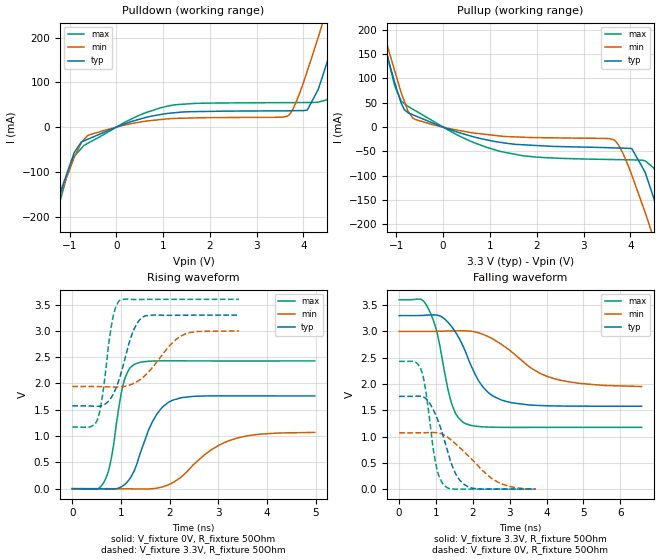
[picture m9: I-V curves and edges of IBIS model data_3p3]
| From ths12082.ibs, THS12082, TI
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|   data_3p3 Model
[Model]   data_3p3
Model_type   Output
Polarity   Non-Inverting
Vmeas = 1.65
Vref = 1.65
Cref = 2pF
Rref = 50
|   typ   min   max
|   (nom PVT)   (fast PVT)   (slow PVT)
C_comp   1.924e-12   1.903e-12   2.001e-12
|ON state : BUFFER OUTPUT TURNED HIGH
|C_comp   1.924e-12   1.903e-12   2.001e-12
|OFF state: BUFFER OUTPUT TURNED LOW
|C_comp   1.784e-12   1.775e-12   1.813e-12
| Where nom  PVT is Nominal Process, 3.3V, 27C
|   Fast PVT is Strong Process,  3.6V, -55C
|   Slow PVT is Weak Process,   3V, 125C
[Voltage Range]   3.3   3   3.6
|Ambient Temperature   25   125   -55
|Junction Temperature
[Temperature Range]   27   125   -55
[Pullup Reference]   3.3   3   3.6
[Pulldown Reference]   0   0   0
[Power Clamp Reference]   3.3   3   3.6
[GND Clamp Reference]   0   0   0
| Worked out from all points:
|   slope of the pulldown table from 0 to 0.495 V, typ, clamps not added: 28 ohm
|   slope of the pullup table from 0 to 0.495 V, typ, clamps not added: 31.6 ohm
|   falling waveform, V_fixture 3.3V, R_fixture 50Ohm: 20-80 % time 746ps typ, 1.26ns min, 438ps max; typ from 3.3 V to 1.58 V
|   rising waveform, V_fixture 0V, R_fixture 50Ohm: 20-80 % time 454ps typ, 853ps min, 253ps max; typ from 0 V to 1.76 V
|   rising waveform, V_fixture 3.3V, R_fixture 50Ohm: 20-80 % time 333ps typ, 577ps min, 204ps max; typ from 1.58 V to 3.3 V
|   falling waveform, V_fixture 0V, R_fixture 50Ohm: 20-80 % time 503ps typ, 947ps min, 288ps max; typ from 1.76 V to 0 V
[Pulldown]
|   Voltage   I(typ)   I(min)   I(max)
-3.3V     -923.6mA   -847.5mA   -1.036A
-1.67V    -308.9mA   -293.9mA   -354.5mA
-1.372V   -205.5mA   -201.5mA   -230.4mA
-896.4mV  -56.13mA   -66.47mA   -64.48mA
-591mV    -26.14mA   -17.73mA   -34.96mA
1.098V    30.73mA    18.6mA     46.91mA
3.66V     36.44mA    24.72mA    54.7mA
4.082V    38.22mA    125.7mA    54.91mA
4.468V    133mA      252.2mA    60.08mA
4.662V    201.8mA    318.6mA    95.82mA
5.062V    345.8mA    460.1mA    239.3mA
6.6V      931.7mA    1.025A     847.3mA
[Pullup]
|   Voltage   I(typ)   I(min)   I(max)
-3.3V     970.9mA    949.6mA    1.007A
-1.325V   196.3mA    214.4mA    194.4mA
-1.03V    89.27mA    113.7mA    83.04mA
-896.4mV  48.97mA    70.33mA    53.32mA
-591mV    23.07mA    15.51mA    33.59mA
1.246V    -31.57mA   -18.54mA   -50.45mA
3.645V    -42.63mA   -26.12mA   -66.6mA
4.033V    -44.37mA   -98.86mA   -67.28mA
4.468V    -136.4mA   -219.7mA   -81.29mA
4.691V    -208.1mA   -289.2mA   -134.2mA
4.871V    -266.7mA   -346.1mA   -198.4mA
6.6V      -907.1mA   -928.5mA   -902.6mA
[Ramp]
R_load = 50
|   typ   min   max
dV/dt_r   1.05827/4.53296e-10   0.642059/8.46681e-10   1.4574/2.51992e-10
dV/dt_f   1.03452/7.42275e-10   0.633874/1.27285e-09   1.45583/4.37549e-10
[Falling Waveform]
V_fixture = 3.3V
V_fixture_min = 3V
V_fixture_max = 3.6V
R_fixture = 50Ohm
|   Time   V(typ)   V(min)   V(max)
0s        3.3V       3V         3.6V
578ps     3.301V     3V         3.613V
764ps     3.31V      3V         3.471V
1.028ns   3.31V      3.001V     2.979V
1.42ns    3.093V     3.008V     1.638V
1.776ns   2.652V     3.01V      1.253V
2.252ns   1.961V     2.95V      1.185V
2.802ns   1.688V     2.74V      1.174V
4.238ns   1.582V     2.095V     1.174V
6.578ns   1.576V     1.951V     1.174V
[Rising Waveform]
V_fixture = 0V
V_fixture_min = 0V
V_fixture_max = 0V
R_fixture = 50Ohm
|   Time   V(typ)   V(min)   V(max)
0s        1.442nV    2.279nV    1.191nV
502ps     -916.8uV   187.4uV    -8.712mV
664ps     -5.071mV   244.1uV    149.2mV
808ps     -9.166mV   -32.17uV   607.8mV
1.042ns   55.58mV    -1.81mV    1.973V
1.28ns    359.4mV    -4.919mV   2.368V
1.648ns   1.278V     -129.3uV   2.426V
2.032ns   1.671V     98.78mV    2.431V
3.188ns   1.765V     903.7mV    2.429V
4.976ns   1.764V     1.07V      2.429V
[Rising Waveform]
V_fixture = 3.3V
V_fixture_min = 3V
V_fixture_max = 3.6V
R_fixture = 50Ohm
|   Time   V(typ)   V(min)   V(max)
0s        1.576V     1.943V     1.174V
374ps     1.571V     1.944V     1.175V
514ps     1.566V     1.942V     1.31V
614ps     1.582V     1.939V     1.731V
822ps     1.765V     1.933V     3.2V
974ps     2.114V     1.935V     3.579V
1.24ns    2.972V     1.992V     3.598V
1.444ns   3.262V     2.112V     3.598V
2.228ns   3.298V     2.901V     3.6V
3.422ns   3.3V       3V         3.6V
[Falling Waveform]
V_fixture = 0V
V_fixture_min = 0V
V_fixture_max = 0V
R_fixture = 50Ohm
|   Time   V(typ)   V(min)   V(max)
0s        1.764V     1.07V      2.429V
422ps     1.766V     1.07V      2.422V
604ps     1.763V     1.071V     2.253V
718ps     1.725V     1.073V     1.888V
1ns       1.396V     1.074V     460.7mV
1.272ns   823.7mV    1.007V     41.44mV
1.54ns    284.4mV    855.9mV    -716uV
1.852ns   50.68mV    649mV      695.3uV
2.654ns   1.493mV    140.8mV    119.3uV
3.702ns   234.5uV    2.611mV    124.3uV
